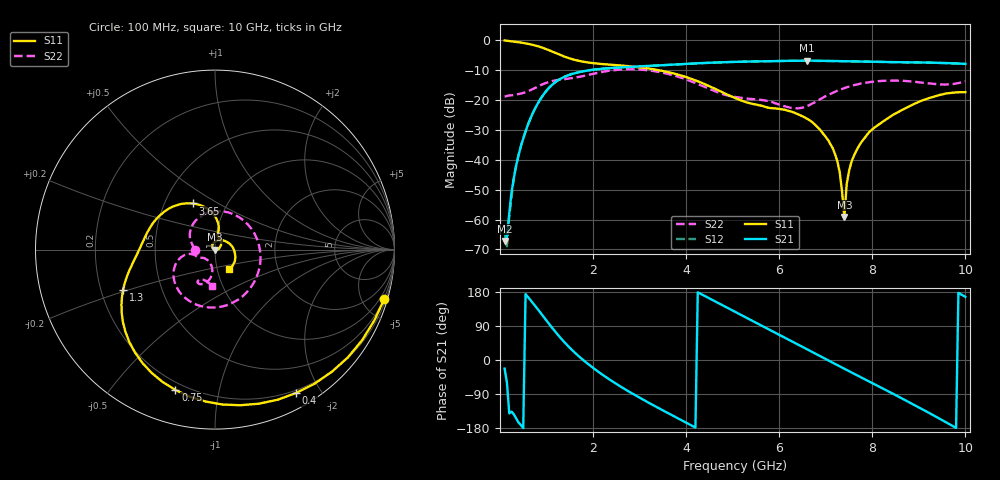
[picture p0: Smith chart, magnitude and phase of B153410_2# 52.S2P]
!  2-Port S-parameters saved by WinCal
! VAR MeasName=S-Parameters (CALIBRATED_DATA) read from VNA (N5245A)
! VAR MeasDate=2016-12-23 10:02:06
! VAR NAME=B153410_2# 52
! VAR FILENAME=B153410_2# 52.S2P
! VAR DATE=2016-12-23 10:02:06
! VAR PHYS_PORTS=1,2
# Hz S DB R 50
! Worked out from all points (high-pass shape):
!   199 points, 100 MHz to 10 GHz, reference 50 ohm
!   highest |S21| = -6.91 dB at 6.6 GHz (marker M1); lowest = -67.2 dB at 100 MHz (marker M2)
!   |S21| within 3 dB of the highest: 2.019 GHz to end of sweep
!   lowest |S11| = -59.2 dB at 7.4 GHz (marker M3), VSWR 1.00, Z = 49.9 - j0.096 ohm
!   |S11| at or under -10 dB: 3.383 GHz to end of sweep
!   |S22| runs from -22.9 to -9.8 dB; largest |S21 - S12| = 0.0029
!   S11 on the Smith chart (normalised r, x): 100 MHz: 0.44, -7.01; 400 MHz: 0.17, -1.70; 750 MHz: 0.16, -0.74; 1.3 GHz: 0.29, -0.19; 3.65 GHz: 0.69, +0.39; 10 GHz: 1.13, -0.26
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1e8  -0.15 -16.2  -67.18 -22.7  -64.02 57.0  -18.89 -179.8
1.5e8  -0.25 -23.9  -65.79 -59.9  -68.90 -68.8  -18.69 178.8
3e8  -0.52 -46.3  -46.09 -143.9  -45.74 -146.3  -18.33 173.9
4e8  -0.75 -60.5  -38.55 -165.1  -38.27 -165.2  -18.07 170.7
7.5e8  -1.81 -105.8  -23.08 143.8  -22.98 144.2  -16.05 153.0
1.3e9  -5.02 -156.1  -12.99 58.5  -12.96 58.5  -13.25 78.0
1.75e9  -7.14 -175.6  -10.59 3.9  -10.56 3.8  -12.18 6.0
2.5e9  -8.41 159.7  -9.24 -63.0  -9.23 -63.2  -9.98 -78.4
3.4e9  -10.04 125.8  -8.50 -126.4  -8.51 -126.4  -10.63 -138.4
3.65e9  -10.87 116.0  -8.29 -142.7  -8.30 -142.8  -11.49 -150.2
5.05e9  -19.40 79.4  -7.31 127.0  -7.33 127.1  -19.04 -161.8
5.85e9  -22.77 76.8  -7.07 76.3  -7.07 76.4  -20.75 -150.3
6.6e9  -26.35 44.2  -6.91 28.2  -6.94 28.2  -22.08 -110.6
6.7e9  -27.34 38.3  -6.91 21.7  -6.94 21.8  -21.30 -105.4
7.2e9  -38.17 -1.1  -7.02 -10.4  -7.03 -10.3  -17.28 -97.0
7.3e9  -44.24 -13.7  -7.06 -16.8  -7.06 -16.6  -16.63 -97.9
7.4e9  -59.16 -119.2  -7.09 -23.0  -7.09 -23.0  -16.08 -98.8
7.45e9  -48.13 -171.5  -7.09 -26.3  -7.11 -26.3  -15.80 -99.5
7.6e9  -38.85 159.0  -7.13 -35.8  -7.15 -35.7  -15.11 -101.6
8.35e9  -26.03 77.9  -7.37 -83.2  -7.38 -83.0  -13.56 -113.8
9.3e9  -19.04 -9.0  -7.58 -145.2  -7.61 -145.0  -14.64 -115.6
1e10  -17.43 -55.5  -8.00 166.6  -8.00 166.9  -13.83 -94.8
